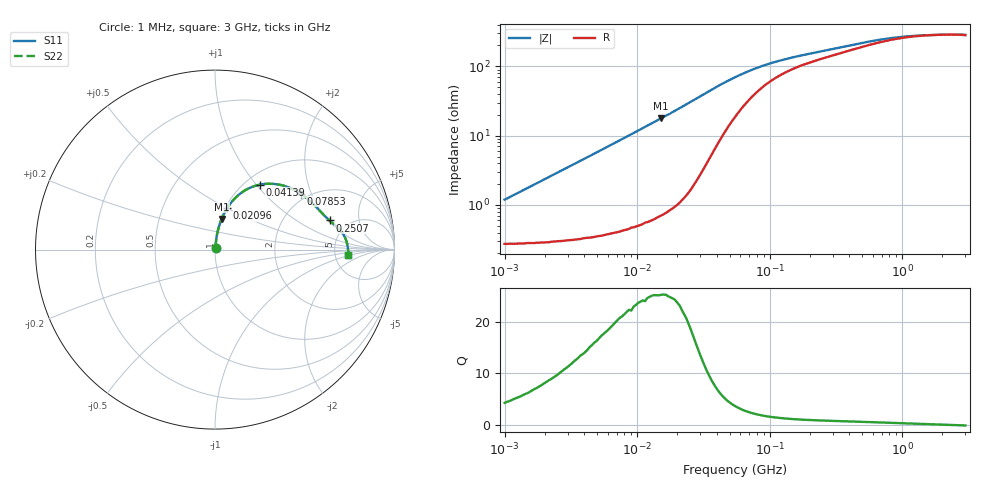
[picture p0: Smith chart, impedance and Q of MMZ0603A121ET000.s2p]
! S-Parameter Data Generated by TDK Corporation
! Copyright(C) 2025 TDK Corporation.
! All Rights Reserved.
! TDK P/N: MMZ0603A121ET000 (Chip Bead)
! Property: |Z|=120ohm at 100MHz
! Size(LxWxT): 0.6x0.3x0.3mm
! Model Type: s2p (Touchstone File Format Version 1.0)
! Frequency: DC=Yes Start=1MHz Stop=3000MHz 202points Log-sweep
! Model Generated on Feb. 6, 2025
! Terms and conditions regarding TDK Simulation Models:
! 1)This simulation model is being provided solely for informational
!  purposes. Please refer to the specifications of the products in
!  terms of detailed characteristics of such products.
! 2)In no event shall TDK Corporation of any of its subsidiaries be
!  liable for any loss or damage arising, directly or indirectly,
!  from any information contained in this simulation model, including,
!  but not limited to loss or damages arising from any inaccuracies,
!  omissions or errors in connection with such information.
! 3)Any and all copyrights on this simulation model are owned by
!  TDK Corporation.  Duplication or redistribution of this simulation
!  model without prior written permission from TDK Corporation
!  is prohibited.
! 4)This simulation model is subject to any modification or change
!  without any prior notice.
! 5)Neither TDK Corporation nor any of its subsidiaries shall make any
!  warranty, express or implied, including but not limited to the
!  correctness, implied warranties of merchantability and fitness for
!  a particular purpose with respect to this simulation models.
! 6)The use of this simulation model shall be deemed to have consented
!  to the terms and conditions hereof.
! Port Assignments:
!  1 ---@@@--- 2
! Applicable Conditions:
!  Temperature = 25 degC
!  DC Bias Current = 0 A
!  Small Signal Operation
# Hz S MA R 50
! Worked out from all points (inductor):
!   201 points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, 1 MHz to 3 GHz, reference 50 ohm
!   read as one part in series: L = 185 nH near 1.041 MHz
!   highest Q = 25.2 at 15.21 MHz (marker M1), where L = 186 nH
!   self-resonance near 2.106 GHz
!   S11 on the Smith chart (normalised r, x): 1 MHz: 1.01, +0.02; 20.96 MHz: 1.02, +0.50; 41.39 MHz: 1.16, +1.04; 78.53 MHz: 1.82, +1.68; 250.7 MHz: 3.60, +2.07; 3 GHz: 6.63, -0.88
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1000000  0.01191 76.0  0.9972 -0.7  0.9972 -0.7  0.01191 76.0
2139570  0.02488 81.9  0.9968 -1.4  0.9968 -1.4  0.02488 81.9
3900413  0.04506 83.3  0.9957 -2.6  0.9957 -2.6  0.04506 83.3
8017732  0.09205 82.1  0.9915 -5.3  0.9915 -5.3  0.09205 82.1
1.461624e7  0.1672 78.1  0.9793 -9.6  0.9793 -9.6  0.1672 78.1
1.521322e7  0.1739 77.7  0.9779 -10.0  0.9779 -10.0  0.1739 77.7
2.095589e7  0.2399 73.7  0.9605 -13.9  0.9605 -13.9  0.2399 73.7
2.886629e7  0.3281 67.0  0.9224 -19.1  0.9224 -19.1  0.3281 67.0
3.526298e7  0.3909 61.0  0.8796 -22.9  0.8796 -22.9  0.3909 61.0
4.138676e7  0.4396 55.4  0.8329 -25.7  0.8329 -25.7  0.4396 55.4
5.477226e7  0.5106 45.0  0.7342 -29.5  0.7342 -29.5  0.5106 45.0
6.428402e7  0.5411 39.4  0.6755 -30.5  0.6755 -30.5  0.5411 39.4
7.852918e7  0.57 33.2  0.6088 -30.8  0.6088 -30.8  0.57 33.2
9.216659e7  0.5874 28.9  0.5625 -30.3  0.5625 -30.3  0.5874 28.9
1.171891e8  0.6076 23.8  0.5073 -28.9  0.5073 -28.9  0.6076 23.8
2.136344e8  0.648 15.7  0.4153 -25.0  0.4153 -25.0  0.648 15.7
2.507343e8  0.6585 14.3  0.3967 -24.2  0.3967 -24.2  0.6585 14.3
4.75755e8  0.7017 9.3  0.3279 -20.3  0.3279 -20.3  0.7017 9.3
8.005644e8  0.7261 5.6  0.2862 -14.3  0.2862 -14.3  0.7261 5.6
1.45942e9  0.7385 1.9  0.2631 -5.4  0.2631 -5.4  0.7385 1.9
2.359433e9  0.7426 -0.6  0.2575 1.8  0.2575 1.8  0.7426 -0.6
3e9  0.7419 -2.3  0.2604 6.6  0.2604 6.6  0.7419 -2.3
